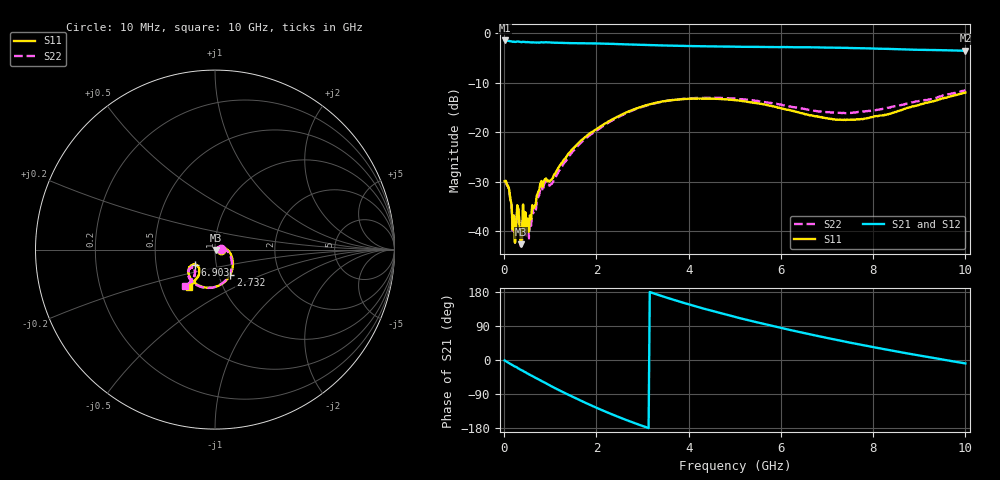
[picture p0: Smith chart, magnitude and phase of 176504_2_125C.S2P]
!  2-Port S-parameters saved by WinCal
! VAR MeasName=S-Parameters (CALIBRATED_DATA) read from VNA (N5242A)
! VAR MeasDate=2017-11-2 17:34:43
! VAR NAME=176504_2_125C
! VAR FILENAME=176504_2_125C.S2P
! VAR DATE=2017-11-2 17:34:43
! VAR PHYS_PORTS=2,3
# Hz S DB R 50
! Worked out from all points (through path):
!   401 points, 10 MHz to 10 GHz, reference 50 ohm
!   highest |S21| = -1.46 dB at 10 MHz (marker M1); lowest = -3.5 dB at 10 GHz (marker M2)
!   lowest |S11| = -42.7 dB at 359.6 MHz (marker M3), VSWR 1.01, Z = 50.7 - j0.245 ohm
!   |S11| at or under -10 dB: start of sweep to end of sweep
!   |S22| runs from -43.0 to -11.5 dB; largest |S21 - S12| = 0.013
!   S11 on the Smith chart (normalised r, x): 10 MHz: 1.07, +0.00; 2.732 GHz: 1.13, -0.33; 6.903 GHz: 0.79, -0.14; 10 GHz: 0.69, -0.31
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1e7  -29.92 0.8  -1.46 -1.1  -1.45 -1.1  -30.08 2.4
1.099e8  -31.61 -27.8  -1.56 -8.6  -1.56 -8.6  -31.73 -29.4
2.098e8  -36.85 -39.8  -1.69 -15.7  -1.69 -15.6  -36.82 -43.9
3.5965e8  -42.68 -19.2  -1.77 -25.9  -1.77 -25.8  -43.02 -32.8
3.84625e8  -41.64 15.5  -1.80 -27.3  -1.80 -27.3  -42.96 7.4
4.5955e8  -36.16 22.0  -1.77 -32.1  -1.77 -32.0  -37.00 17.0
5.34475e8  -40.10 16.4  -1.82 -37.6  -1.82 -37.6  -41.45 7.5
7.5925e8  -31.72 34.7  -1.90 -51.9  -1.90 -51.9  -32.72 32.7
8.5915e8  -29.93 22.6  -1.87 -58.4  -1.87 -58.3  -30.76 18.7
1.009e9  -29.71 12.7  -1.87 -68.5  -1.87 -68.4  -30.56 7.6
1.333675e9  -25.22 7.6  -1.98 -88.2  -1.98 -88.3  -25.87 4.2
1.683325e9  -21.54 -10.6  -2.02 -108.4  -2.02 -108.3  -21.95 -14.2
2.2078e9  -18.18 -36.4  -2.12 -136.8  -2.11 -136.7  -18.39 -38.8
2.732275e9  -15.66 -59.1  -2.27 -162.2  -2.27 -162.0  -15.78 -60.4
3.35665e9  -13.94 -83.1  -2.45 171.2  -2.46 171.3  -13.96 -84.0
4.180825e9  -13.21 -109.6  -2.61 140.6  -2.63 140.9  -13.08 -108.9
5.005e9  -13.51 -130.3  -2.71 113.7  -2.71 114.1  -13.23 -128.1
5.829175e9  -14.78 -143.4  -2.79 89.6  -2.83 90.0  -14.14 -140.1
6.678325e9  -16.66 -144.6  -2.84 66.6  -2.86 67.0  -15.59 -142.7
6.9031e9  -17.06 -143.1  -2.88 60.8  -2.88 61.1  -15.90 -142.1
8.35165e9  -16.27 -123.7  -3.15 26.0  -3.19 26.6  -15.01 -129.0
1e10  -11.98 -124.9  -3.54 -9.1  -3.56 -8.2  -11.52 -129.6
